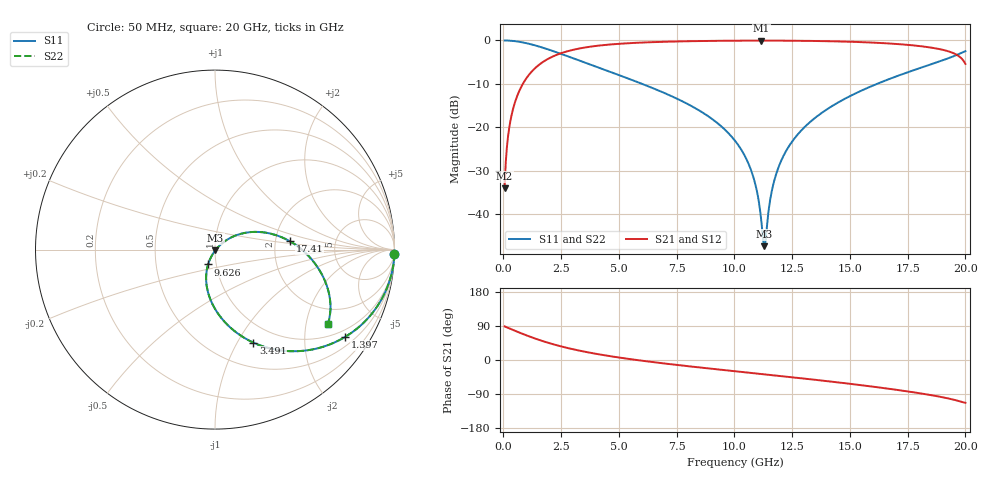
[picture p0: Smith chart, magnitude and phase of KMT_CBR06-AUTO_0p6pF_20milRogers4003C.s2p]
! Data measured by Modelithics Inc. support@modelithics.com 813-866-6335
! KEMET CBR06-AUTO 0.6pF, Pad Width= 0.851mm, Pad Length= 0.64mm, Pad Gap= 0.62mm, 20mil Rogers 4003C substrate Data, January 2022
# hz S ma R 50
! 2 Port Network Data from SP1.SP block
! freq  magS11  angS11  magS21  angS21  magS12  angS12  magS22  angS22
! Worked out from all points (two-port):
!   401 points, 50 MHz to 20 GHz, reference 50 ohm
!   highest |S21| = -0.04 dB at 11.17 GHz (marker M1); lowest = -34.1 dB at 50 MHz (marker M2)
!   |S21| within 3 dB of the highest: 2.443 GHz to 19.53 GHz (17.08 GHz wide, 156 % of centre)
!   lowest |S11| = -47.4 dB at 11.27 GHz (marker M3), VSWR 1.01, Z = 50.2 - j0.357 ohm
!   |S11| at or under -10 dB: 5.997 GHz to 16.18 GHz (10.18 GHz wide, 91.8 % of centre)
!   |S22| runs from -47.4 to 0.0 dB; largest |S21 - S12| = 0
!   S11 on the Smith chart (normalised r, x): 50 MHz: 1, -88; 1.397 GHz: 0.76, -3.12; 3.491 GHz: 0.77, -1.17; 9.626 GHz: 0.91, -0.15; 17.41 GHz: 2.42, +0.27; 20 GHz: 1.41, -2.68
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5e7  0.9998 -1.3  0.01974 88.7  0.01974 88.7  0.9998 -1.3
2.495e8  0.9951 -6.5  0.0981 83.5  0.0981 83.5  0.9951 -6.5
4.49e8  0.9845 -11.6  0.1748 78.4  0.1748 78.4  0.9845 -11.6
8.48e8  0.9477 -21.5  0.3186 68.5  0.3186 68.5  0.9477 -21.5
1.396625e9  0.8731 -33.9  0.4865 56.1  0.4865 56.1  0.8731 -33.9
3.391625e9  0.5731 -66.4  0.8175 23.4  0.8175 23.4  0.5731 -66.4
3.491375e9  0.5604 -67.6  0.8262 22.2  0.8262 22.2  0.5604 -67.6
6.73325e9  0.2635 -96.9  0.9617 -7.5  0.9617 -7.5  0.2635 -96.9
9.626e9  0.09153 -114.9  0.992 -27.1  0.992 -27.1  0.09153 -114.9
1.0025e10  0.06974 -116.7  0.9937 -29.6  0.9937 -29.6  0.06974 -116.7
1.077312e10  0.02908 -116.9  0.9954 -34.4  0.9954 -34.4  0.02908 -116.9
1.10225e10  0.01564 -111.5  0.9956 -36.0  0.9956 -36.0  0.01564 -111.5
1.117212e10  0.007964 -97.1  0.9956 -37.0  0.9956 -37.0  0.007964 -97.1
1.127188e10  0.004245 -56.7  0.9956 -37.6  0.9956 -37.6  0.004245 -56.7
1.137162e10  0.005793 7.3  0.9955 -38.2  0.9955 -38.2  0.005793 7.3
1.167088e10  0.02125 38.5  0.9952 -40.2  0.9952 -40.2  0.02125 38.5
1.197012e10  0.03797 41.3  0.9945 -42.1  0.9945 -42.1  0.03797 41.3
1.336662e10  0.1203 36.2  0.9871 -51.3  0.9871 -51.3  0.1203 36.2
1.670825e10  0.3594 12.3  0.9225 -76.1  0.9225 -76.1  0.3594 12.3
1.74065e10  0.4207 6.2  0.8942 -82.1  0.8942 -82.1  0.4207 6.2
1.910225e10  0.6018 -12.1  0.7703 -99.4  0.7703 -99.4  0.6018 -12.1
2e10  0.7528 -33.3  0.5366 -113.0  0.5366 -113.0  0.7528 -33.3
